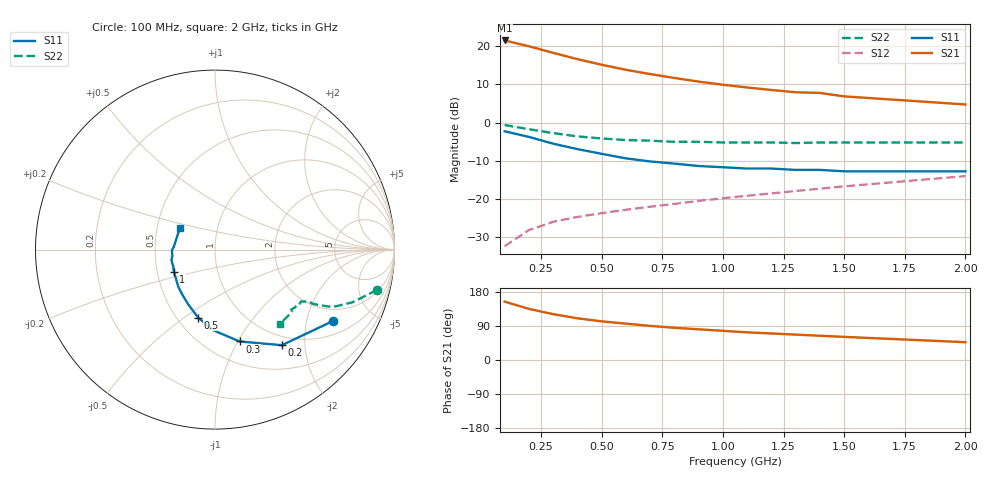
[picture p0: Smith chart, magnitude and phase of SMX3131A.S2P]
! HSMX-3131 Common Emitter
! Vce=10V Ic=5ma
# ghz s ma r 50
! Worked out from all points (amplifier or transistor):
!   16 points, 100 MHz to 2 GHz, reference 50 ohm
!   highest |S21| = 21.5 dB at 100 MHz (marker M1)
!   |S21| within 3 dB of that: start of sweep to 285.5 MHz
!   unconditionally stable (mu >= 1): 894.1 MHz to end of sweep
!   at 300 MHz: K = 0.24, MSG = 22.2 dB, |S12| = -26.0 dB
!   at 900 MHz: K = 1.00, MAG = 15.4 dB, |S12| = -20.5 dB
!   at 2 GHz: K = 1.01, MAG = 8.9 dB, |S12| = -14.0 dB
!   S11 on the Smith chart (normalised r, x): 100 MHz: 1.49, -2.91; 200 MHz: 0.85, -1.57; 300 MHz: 0.71, -1.02; 500 MHz: 0.63, -0.56; 1 GHz: 0.61, -0.16; 2 GHz: 0.66, +0.17
0.1  0.77 -31.0  11.95 154.0  0.024 154.0  0.93 -14.0
0.2  0.65 -55.0  10.03 135.0  0.039 135.0  0.82 -21.0
0.3  0.53 -75.0  8.22 121.0  0.05 121.0  0.73 -26.0
0.4  0.45 -91.0  6.8 110.0  0.058 110.0  0.66 -28.0
0.5  0.39 -104.0  5.74 102.0  0.065 102.0  0.62 -29.0
0.6  0.34 -116.0  4.93 96.0  0.072 96.0  0.59 -29.0
0.7  0.31 -126.0  4.33 90.0  0.079 90.0  0.58 -30.0
0.8  0.29 -135.0  3.85 85.0  0.086 85.0  0.56 -31.0
0.9  0.27 -144.0  3.45 81.0  0.094 81.0  0.56 -33.0
1  0.26 -152.0  3.14 77.0  0.102 77.0  0.55 -34.0
1.1  0.25 -159.0  2.89 73.0  0.11 73.0  0.55 -35.0
1.2  0.25 -166.0  2.68 70.0  0.118 70.0  0.55 -36.0
1.3  0.24 -172.0  2.5 67.0  0.127 67.0  0.54 -38.0
1.4  0.24 -179.0  2.45 64.0  0.136 64.0  0.55 -39.0
1.5  0.23 176.0  2.21 61.0  0.146 61.0  0.55 -41.0
2  0.23 148.0  1.73 47.0  0.199 47.0  0.55 -49.0
